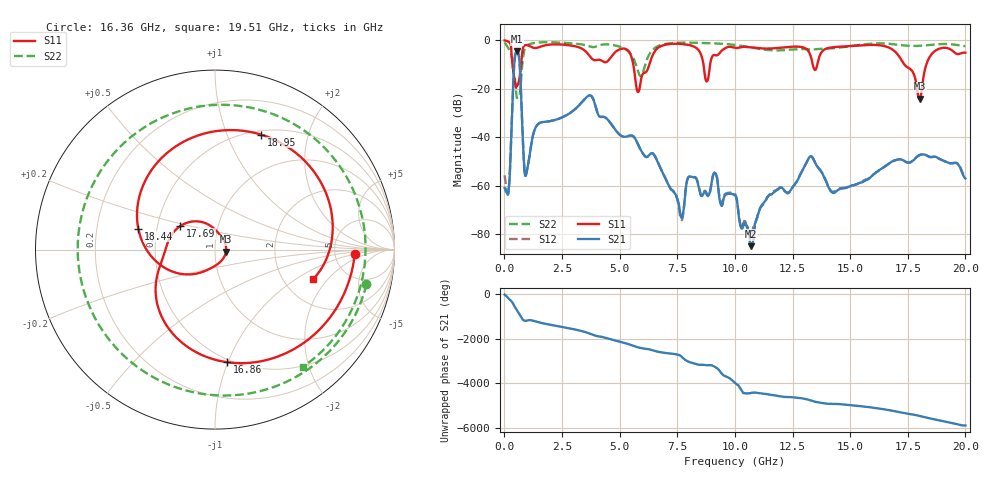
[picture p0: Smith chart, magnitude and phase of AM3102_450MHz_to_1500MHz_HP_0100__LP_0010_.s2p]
!Agilent Technologies,E8364B,MY43040894,A.07.50.67
!Agilent E8364B: A.07.50.67
!Date: Thursday, January 11, 2018 05:35:19
!Correction: S11(Full 2 Port(1,2))
!S21(Full 2 Port(1,2))
!S12(Full 2 Port(1,2))
!S22(Full 2 Port(1,2))
!S2P File: Measurements: S11, S21, S12, S22:
# Hz S  dB  R 50
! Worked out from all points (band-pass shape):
!   1601 points, 10 MHz to 20 GHz, reference 50 ohm
!   highest |S21| = -4.52 dB at 534.7 MHz (marker M1); lowest = -85.0 dB at 10.68 GHz (marker M2)
!   |S21| within 3 dB of the highest: 449.4 MHz to 642.3 MHz (192.9 MHz wide, 35.3 % of centre)
!   lowest |S11| = -24.1 dB at 18.01 GHz (marker M3), VSWR 1.13, Z = 56.5 - j1.24 ohm
!   |S11| at or under -10 dB: 349.6 MHz to 725.9 MHz (376.2 MHz wide, 70 % of centre); 5.592 GHz to 6.288 GHz (696.3 MHz wide, 11.7 % of centre); 17.36 GHz to 18.31 GHz (950 MHz wide, 5.33 % of centre)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
!   |S22| runs from -23.8 to -0.8 dB; largest |S21 - S12| = 0.0021
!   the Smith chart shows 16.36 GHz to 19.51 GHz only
!   S11 on the Smith chart (normalised r, x): 16.36 GHz: 7.94, -0.88; 16.86 GHz: 0.48, -0.99; 17.69 GHz: 0.66, +0.18; 18.44 GHz: 0.39, +0.11; 18.95 GHz: 0.54, +1.33; 19.51 GHz: 2.88, -1.42
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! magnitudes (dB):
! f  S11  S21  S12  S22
! 10 MHz  -0.1  -60.9  -55.7  -0.9
! 197.4 MHz  -0.7  -60.6  -60.6  -3.8
! 534.7 MHz  -18.5  -4.5  -4.5  -23.4
! 947 MHz  -1.9  -55.1  -55.2  -2.5
! 3.346 GHz  -3.4  -25.7  -25.7  -1.7
! 5.807 GHz  -21.3  -43.2  -43.2  -13.0
! 6.682 GHz  -3.0  -50.9  -50.8  -2.3
! 7.669 GHz  -1.5  -73.0  -74.1  -1.0
! 8.056 GHz  -2.0  -56.2  -56.2  -1.0
! 8.781 GHz  -17.0  -63.6  -63.6  -1.1
! 10.01 GHz  -3.1  -64.0  -63.4  -1.9
! 10.68 GHz  -2.9  -85.0  -80.0  -2.9
! 13.34 GHz  -8.4  -48.1  -48.1  -3.8
! 16.36 GHz  -2.2  -53.0  -52.9  -1.3
! 16.68 GHz  -3.0  -50.9  -50.9  -1.4
! 16.86 GHz  -4.0  -49.8  -49.8  -1.6
! 17.69 GHz  -12.6  -49.9  -49.9  -2.3
! 18.01 GHz  -24.1  -47.4  -47.3  -2.3
! 18.44 GHz  -7.1  -48.1  -48.1  -1.9
! 18.95 GHz  -3.2  -49.3  -49.3  -1.6
! 19.51 GHz  -4.9  -50.6  -50.5  -1.8
! 20 GHz  -5.1  -57.0  -57.1  -2.4
